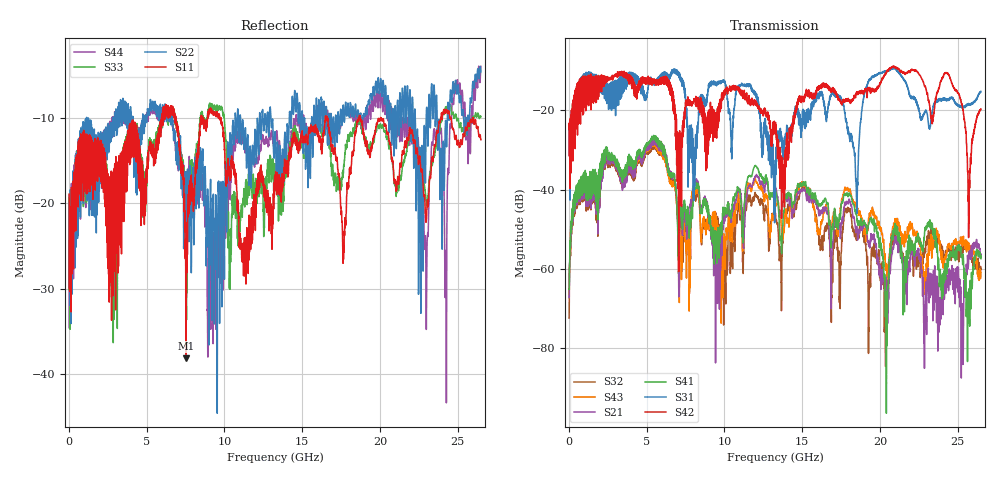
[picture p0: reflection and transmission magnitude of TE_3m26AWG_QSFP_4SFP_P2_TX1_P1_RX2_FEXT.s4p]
!Agilent Technologies,N5222A,MY51421691,A.10.00.00
!Agilent N5222A: A.10.00.00
!Date: Friday, January 30, 2015 12:36:39
!Correction: S11(Full 4 Port(1,2,3,4))
!S12(Full 4 Port(1,2,3,4))
!S13(Full 4 Port(1,2,3,4))
!S14(Full 4 Port(1,2,3,4))
!S21(Full 4 Port(1,2,3,4))
!S22(Full 4 Port(1,2,3,4))
!S23(Full 4 Port(1,2,3,4))
!S24(Full 4 Port(1,2,3,4))
!S31(Full 4 Port(1,2,3,4))
!S32(Full 4 Port(1,2,3,4))
!S33(Full 4 Port(1,2,3,4))
!S34(Full 4 Port(1,2,3,4))
!S41(Full 4 Port(1,2,3,4))
!S42(Full 4 Port(1,2,3,4))
!S43(Full 4 Port(1,2,3,4))
!S44(Full 4 Port(1,2,3,4))
!S4P File: Measurements: <S11,S12,S13,S14>,
!<S21,S22,S23,S24>,
!<S31,S32,S33,S34>,
!<S41,S42,S43,S44>:
# Hz S  dB  R 50.0
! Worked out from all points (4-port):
!   2650 points, 10 MHz to 26.5 GHz, reference 50 ohm
!   strongest paths, dB at 10 MHz, 6.63 GHz, 13.26 GHz, 19.88 GHz, 26.5 GHz:
!     S42: -24.7, -16.2, -25.1, -14.1, -19.7
!     S31: -25.0, -10.3, -36.2, -10.7, -15.2
!     S41: -65.2, -35.8, -40.3, -51.6, -57.4
!     S21: -67.2, -36.0, -39.4, -57.8, -56.3
!     S43: -66.4, -38.5, -43.6, -48.9, -60.9
!     S32: -72.4, -37.7, -44.9, -59.0, -60.1
!   lowest |S11| = -38.1 dB at 7.52 GHz (marker M1), VSWR 1.03, Z = 51.2 + j0.312 ohm
!   |S11| at or under -10 dB: start of sweep to 5.956 GHz; 9.72 GHz to 16.5 GHz (6.776 GHz wide, 51.7 % of centre); 20.05 GHz to 23.92 GHz (3.866 GHz wide, 17.6 % of centre)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
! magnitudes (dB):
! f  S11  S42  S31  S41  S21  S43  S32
! 10 MHz  -18.9  -24.7  -25.0  -65.2  -67.2  -66.4  -72.4
! 2.35 GHz  -14.6  -11.5  -13.0  -32.0  -33.4  -32.4  -34.0
! 7.52 GHz  -38.1  -18.9  -19.8  -45.4  -46.5  -54.9  -51.6
! 18.49 GHz  -11.1  -15.5  -41.7  -46.3  -50.3  -44.5  -52.3
! 19.59 GHz  -12.2  -15.3  -11.4  -47.7  -52.2  -45.5  -54.8
! 22.98 GHz  -22.1  -14.8  -20.1  -49.2  -75.2  -58.7  -53.0
! 26.5 GHz  -12.6  -19.7  -15.2  -57.4  -56.3  -60.9  -60.1
